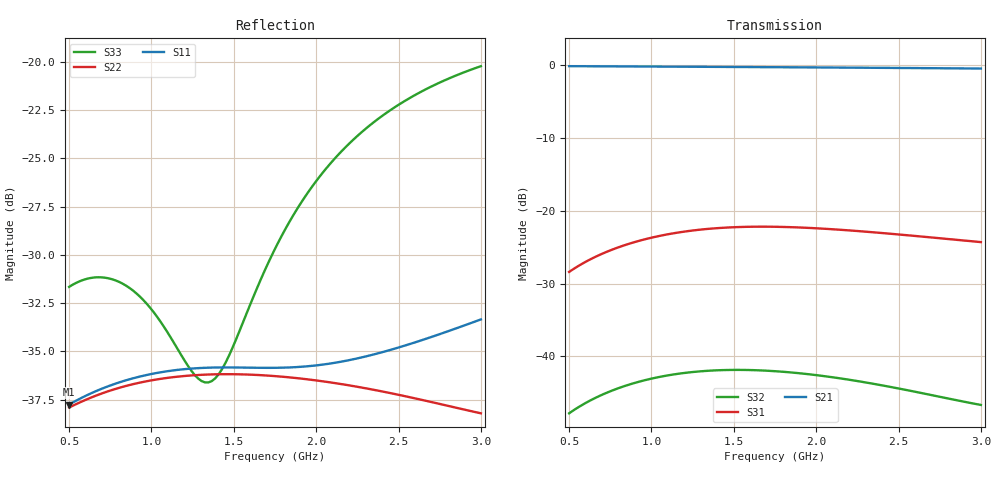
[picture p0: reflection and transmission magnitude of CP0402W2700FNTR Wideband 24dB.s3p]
!	AVX THIN FILM OPERATION
!	CP0402 WIDEBAND HIGH DIRECTIVITY  COUPLER
!	P/N CP0402W2700FNTR
! 	3 April 2012
# hz S ma R 50
! 3 Port Network Data from data block
! freq  magS11  angS11  magS12  angS12  magS13  angS13
!  magS21  angS21
!  magS22  angS22  magS23  angS23
!  magS31  angS31  magS32  angS32
!  magS33  angS33
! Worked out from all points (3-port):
!   121 points, 500 MHz to 3 GHz, reference 50 ohm
!   strongest paths, dB at 500 MHz, 991.7 MHz, 1.617 GHz, 2.242 GHz, 3 GHz:
!     S21: -0.1, -0.2, -0.2, -0.3, -0.4
!     S31: -28.4, -23.7, -22.2, -22.8, -24.3
!     S32: -47.8, -43.1, -41.9, -43.4, -46.7
!   lowest |S11| = -37.8 dB at 500 MHz (marker M1), VSWR 1.03, Z = 51.3 + j0.246 ohm
!   |S11| at or under -10 dB: start of sweep to end of sweep
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5e8  0.01295 10.7  0.9864 -3.6  0.03806 66.0
     0.9864 -3.6  0.01272 9.7  0.004066 71.9
     0.03806 66.0  0.004066 71.9  0.02614 -91.1
6.875e8  0.01417 9.2  0.9843 -4.8  0.04997 57.4
         0.9843 -4.8  0.01378 8.2  0.005372 65.0
         0.04997 57.4  0.005372 65.0  0.02768 -109.6
8.666667e8  0.01506 6.6  0.9821 -6.0  0.05956 49.5
            0.9821 -6.0  0.01455 5.6  0.006416 58.6
            0.05956 49.5  0.006416 58.6  0.02597 -122.1
1.2625e9  0.01608 0.1  0.9772 -8.6  0.07357 33.3
          0.9772 -8.6  0.01543 -1.6  0.007837 45.6
          0.07357 33.3  0.007837 45.6  0.01545 -114.7
1.345833e9  0.01614 -1.1  0.9761 -9.2  0.07523 30.3
            0.9761 -9.2  0.01549 -3.2  0.007971 43.1
            0.07523 30.3  0.007971 43.1  0.01478 -101.1
1.45e9  0.01616 -2.4  0.9747 -9.9  0.0767 26.6
        0.9747 -9.9  0.01552 -5.3  0.008064 40.3
        0.0767 26.6  0.008064 40.3  0.01663 -83.5
1.7625e9  0.01613 -4.8  0.9703 -11.9  0.0777 16.9
          0.9703 -11.9  0.01533 -11.9  0.007899 33.6
          0.0777 16.9  0.007899 33.6  0.03361 -67.0
1.991667e9  0.01635 -5.1  0.9669 -13.4  0.076 11.3
            0.9669 -13.4  0.01497 -17.2  0.00746 30.5
            0.076 11.3  0.00746 30.5  0.0486 -71.4
2.2625e9  0.01711 -5.3  0.9627 -15.1  0.07251 6.3
          0.9627 -15.1  0.01437 -23.9  0.006737 29.2
          0.07251 6.3  0.006737 29.2  0.06503 -80.0
3e9  0.02152 -11.6  0.95 -19.8  0.06101 -0.0
     0.95 -19.8  0.01229 -48.2  0.004643 42.8
     0.06101 -0.0  0.004643 42.8  0.09756 -101.9
